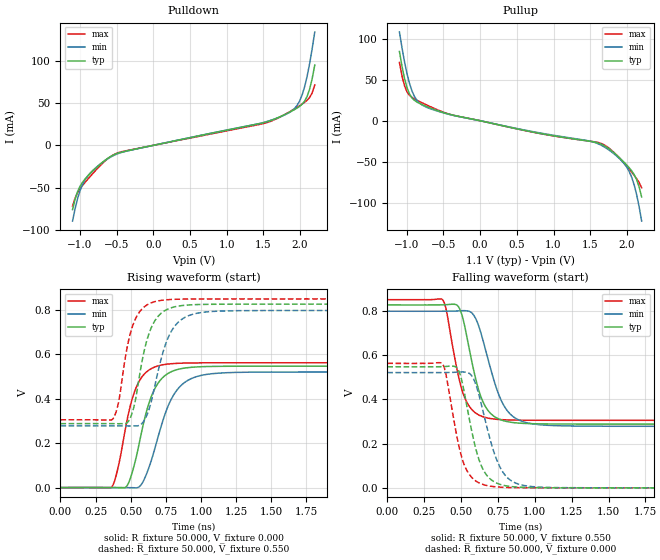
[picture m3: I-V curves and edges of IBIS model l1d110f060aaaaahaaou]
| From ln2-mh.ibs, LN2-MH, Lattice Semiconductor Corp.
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|   Model l1d110f060aaaaahaaou
[Model] l1d110f060aaaaahaaou
Model_type Output
Polarity   Non-Inverting
Enable   Active-High
Vmeas =  0.550V
Cref =  20.000pF
Rref =  50.000
Vref =  0.600V
C_comp   2.000pF   1.500pF   2.500pF
[Temperature Range]   25.000   0.125k   -40.000
[Voltage Range]   1.100V   1.070V   1.130V
[C Comp Corner]
C_comp   2.000pF   1.500pF   2.500pF
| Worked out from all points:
|   slope of the pulldown table from 0 to 0.165 V, typ, clamps not added: 54.8 ohm
|   slope of the pullup table from 0 to 0.165 V, typ, clamps not added: 49.8 ohm
|   rising waveform, R_fixture 50.000, V_fixture 0.000: 20-80 % time 137ps typ, 168ps min, 121ps max; typ from 0 V to 0.547 V
|   rising waveform, R_fixture 50.000, V_fixture 0.550: 20-80 % time 111ps typ, 136ps min, 99.4ps max; typ from 0.288 V to 0.826 V
|   falling waveform, R_fixture 50.000, V_fixture 0.550: 20-80 % time 116ps typ, 145ps min, 104ps max; typ from 0.826 V to 0.288 V
|   falling waveform, R_fixture 50.000, V_fixture 0.000: 20-80 % time 112ps typ, 134ps min, 103ps max; typ from 0.547 V to 0 V
[Pulldown]
|Voltage   I(typ)   I(min)   I(max)
-1.1V     -76.12mA   -89.68mA   -72.01mA
-1.032V   -54.89mA   -63.31mA   -56.1mA
-930mV    -39.97mA   -40.86mA   -43.93mA
-794mV    -27.89mA   -27.32mA   -30.51mA
-556mV    -12.02mA   -12.75mA   -11.86mA
-318mV    -5.813mA   -5.931mA   -5.496mA
1.518V    27.25mA    27.47mA    26.2mA
1.892V    40.87mA    41.2mA     41.62mA
1.994V    46.21mA    52.59mA    47.06mA
2.062V    52.43mA    69.57mA    51.01mA
2.13V     66.65mA    96.98mA    56.74mA
2.2V      95.12mA    134.3mA    71.6mA
[Pullup]
|Voltage   I(typ)   I(min)   I(max)
-1.1V     84.55mA    108.3mA    71.12mA
-1.064V   65.89mA    88.49mA    54.15mA
-996mV    40.18mA    57.16mA    35.1mA
-928mV    27.8mA     36.06mA    28.38mA
-826mV    21.09mA    21.55mA    23.38mA
-350mV    6.36mA     6.205mA    6.35mA
1.656V    -28.96mA   -30.26mA   -28.06mA
1.894V    -44.87mA   -45.95mA   -45.33mA
2.03V     -57.4mA    -61.9mA    -59.23mA
2.098V    -65.83mA   -78.31mA   -66.71mA
2.132V    -72.05mA   -90.37mA   -70.79mA
2.2V      -93.13mA   -122.5mA   -81.91mA
[Ramp]
| variable   typ   min   max
dV/dt_r   0.328/0.137n   0.312/0.168n   0.337/0.121n
dV/dt_f   0.314/0.124n   0.307/0.165n   0.314/0.105n
R_load = 50.000
[Rising Waveform]
R_fixture = 50.000
V_fixture = 0.000
V_fixture_min = 0.000
V_fixture_max = 0.000
|  time   V(typ)   V(min)   V(max)
0s        1.692uV    8.245uV    473.4nV
362ps     84.1uV     65.4uV     1.097mV
467ps     3.007mV    -208.4uV   280.6mV
524ps     98.39mV    -727.5uV   425.8mV
591ps     288.7mV    30.47mV    506.9mV
676ps     450.7mV    185.8mV    544mV
788ps     521.4mV    397.2mV    557.6mV
928ps     541.3mV    489.8mV    561.1mV
1.238ns   546.3mV    518.3mV    561.9mV
10ns      546.6mV    520.5mV    562mV
[Rising Waveform]
R_fixture = 50.000
V_fixture = 0.550
V_fixture_min = 0.534
V_fixture_max = 0.568
|  time   V(typ)   V(min)   V(max)
0s        287.8mV    277.6mV    304.9mV
372ps     287.9mV    277.7mV    308.5mV
415ps     287.5mV    277.7mV    388.6mV
479ps     294.7mV    277.3mV    644.2mV
528ps     377.1mV    277.6mV    750.9mV
609ps     649.4mV    317.2mV    819.4mV
757ps     801.5mV    660.6mV    845.6mV
906ps     821.8mV    772.4mV    848.9mV
1.256ns   825.7mV    796.3mV    849.6mV
10ns      825.8mV    797.4mV    849.6mV
[Falling Waveform]
R_fixture = 50.000
V_fixture = 0.550
V_fixture_min = 0.534
V_fixture_max = 0.568
|  time   V(typ)   V(min)   V(max)
0s        825.8mV    797.4mV    849.6mV
374ps     826mV      797.4mV    849.5mV
479ps     820.5mV    798.8mV    514.2mV
534ps     699.1mV    799.5mV    392.7mV
599ps     491.9mV    764.2mV    337.8mV
659ps     373.9mV    639.9mV    318.8mV
743ps     314.9mV    443.5mV    309.3mV
883ps     292.8mV    309mV      305.7mV
1.203ns   288.1mV    279.7mV    304.9mV
10ns      287.8mV    277.6mV    304.9mV
[Falling Waveform]
R_fixture = 50.000
V_fixture = 0.000
V_fixture_min = 0.000
V_fixture_max = 0.000
|  time   V(typ)   V(min)   V(max)
0s        546.6mV    520.5mV    562mV
371ps     547.1mV    520.5mV    561.8mV
471ps     542.3mV    522.3mV    234.4mV
525ps     419.3mV    522.7mV    98.49mV
589ps     205.6mV    485.4mV    36.5mV
649ps     83.04mV    344.8mV    15.09mV
743ps     21mV       124mV      4.115mV
863ps     4.387mV    23.64mV    931.6uV
1.114ns   342.3uV    1.562mV    98.18uV
10ns      1.692uV    8.245uV    473.4nV
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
